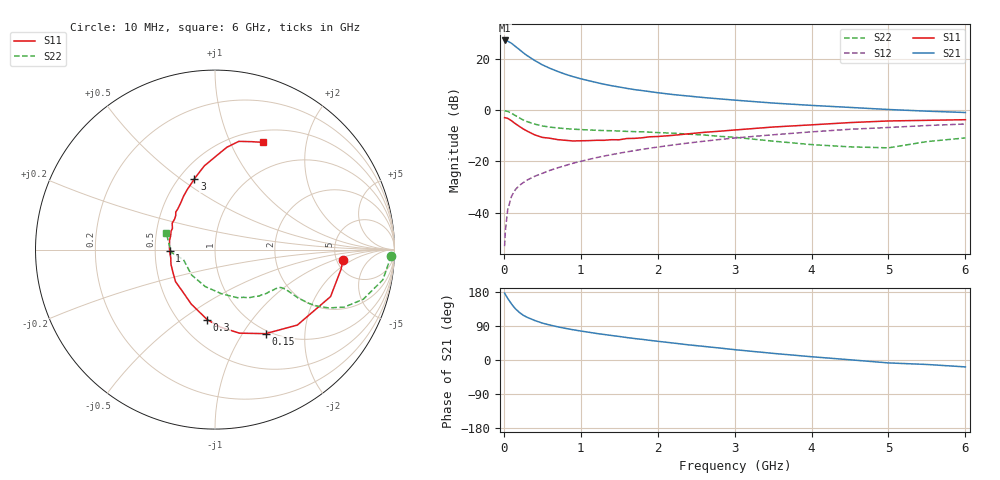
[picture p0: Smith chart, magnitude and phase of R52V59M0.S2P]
! SIEMENS Small Signal Semiconductors
! BFR183
! Si NPN RF Bipolar Junction Transistor in SOT23
! VCE = 2.5 V  IC = 9 mA
! Common Emitter S-Parameters:  May  1996
# GHz  S  MA  R  50
!  f  S11  S21  S12  S22
! GHz  MAG  ANG  MAG  ANG  MAG  ANG  MAG  ANG
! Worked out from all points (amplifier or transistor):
!   36 points, 10 MHz to 6 GHz, reference 50 ohm
!   highest |S21| = 27.3 dB at 10 MHz (marker M1)
!   |S21| within 3 dB of that: start of sweep to 178.5 MHz
!   unconditionally stable (mu >= 1): 790.8 MHz to 2.502 GHz
!   at 250 MHz: K = 0.60, MSG = 25.5 dB, |S12| = -28.4 dB
!   at 1.4 GHz: K = 1.06, MAG = 12.0 dB, |S12| = -17.4 dB
!   at 6 GHz: K = 0.89, MSG = 2.2 dB, |S12| = -5.4 dB
!   S11 on the Smith chart (normalised r, x): 10 MHz: 5.69, -1.37; 150 MHz: 0.95, -1.27; 300 MHz: 0.68, -0.63; 1 GHz: 0.60, -0.01; 3 GHz: 0.59, +0.56; 6 GHz: 0.64, +1.33
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0.01  0.7156 -4.7  23.15 176.6  0.0022 84.8  0.9822 -2.0
0.02  0.7106 -8.9  22.82 172.8  0.0044 82.7  0.9715 -4.2
0.05  0.6952 -22.1  22.45 162.7  0.0113 79.6  0.9503 -10.2
0.1  0.6223 -42.5  20.38 147.8  0.0208 71.9  0.8713 -18.5
0.15  0.5464 -59.0  17.68 135.2  0.0281 66.6  0.7882 -24.0
0.2  0.485 -73.7  15.48 125.9  0.0336 63.5  0.7107 -27.2
0.25  0.4333 -85.9  13.42 118.4  0.0382 61.3  0.6471 -29.0
0.3  0.3927 -96.3  11.77 112.9  0.043 61.6  0.6017 -29.8
0.4  0.3307 -113.7  9.428 104.4  0.0511 61.3  0.5364 -30.2
0.5  0.2947 -128.1  7.742 97.4  0.0584 62.2  0.4933 -29.8
0.6  0.2832 -141.0  6.592 92.2  0.0668 63.0  0.4675 -29.5
0.7  0.2664 -151.7  5.737 87.6  0.0749 63.9  0.4511 -29.4
0.8  0.2585 -161.6  5.06 83.5  0.0831 63.8  0.4368 -29.6
1  0.253 -178.2  4.127 76.5  0.1003 64.6  0.419 -30.3
1.1  0.2547 175.6  3.792 73.4  0.109 64.4  0.412 -31.3
1.6  0.2802 148.3  2.675 59.2  0.1536 62.3  0.3861 -36.9
2.2  0.3233 126.1  2.028 44.8  0.2095 57.8  0.3567 -46.5
3  0.411 106.2  1.578 27.3  0.2866 49.4  0.2962 -64.9
3.5  0.4701 97.3  1.383 17.5  0.3315 43.3  0.2488 -81.5
4.5  0.5739 83.4  1.136 0.6  0.4248 30.9  0.1924 -132.8
5.5  0.6352 71.2  0.96 -11.8  0.5029 18.9  0.244 -176.3
6  0.6536 66.1  0.903 -18.2  0.5382 11.0  0.2876 161.0
